TYPE ConfigChiller :
STRUCT
	Enable:BOOL;
	MFG:SVINT;
	CommType:SVINT;
	Port:STRING;
	TempOffset:SVLREAL;
	MaxLimit:SVLREAL;
	MinLimit:SVLREAL;
	EnableAlarmTolerance:BOOL;
	ToleranceAlarmRange:SVINT;
	ToleranceAlarmTime:SVINT;
END_STRUCT
END_TYPE
